PROGRAM MAIN

VAR
bRun : BOOL := FALSE;
fGaugeValue : REAL := 0.0;
END_VAR

IF bRun THEN

fGaugeValue := fGaugeValue + 0.1;

IF fGaugeValue >= 100.0 THEN
    fGaugeValue := 100.0;
END_IF

ELSE

fGaugeValue := fGaugeValue - 0.1;

IF fGaugeValue <= 0.0 THEN
    fGaugeValue := 0.0;
END_IF

END_IF

END_PROGRAM
